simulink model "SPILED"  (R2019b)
settings: Solver=FixedStepDiscrete  StartTime=0.0  StopTime=inf  FixedStep=0.001  RelTol=1e-3  EnableMultiTasking=on
libraries: c2837xDlib x2, demo_controls x1, simulink x1, c280xlib x1

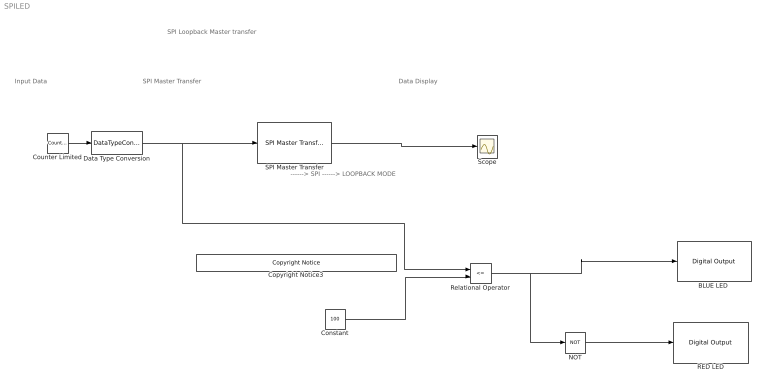
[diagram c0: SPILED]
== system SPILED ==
  note: SPI Loopback Master transfer
  note: Input Data
  note: SPI Master Transfer
  note: ------> SPI ------> LOOPBACK MODE
  note: Data Display
  "BLUE LED " : c2837xDlib/Digital Output  GPIO_Number=GPIO24~GPIO31  GPIO_Bit0=off  GPIO_BIT0_Toggle=off  GPIO_Bit1=off  GPIO_BIT1_Toggle=off  GPIO_Bit2=off  GPIO_BIT2_Toggle=off  GPIO_Bit3=off  GPIO_BIT3_Toggle=off  GPIO_Bit4=off  GPIO_BIT4_Toggle=off  GPIO_Bit5=off  GPIO_BIT5_Toggle=off  GPIO_Bit6=off  GPIO_BIT6_Toggle=off  GPIO_Bit7=on  GPIO_BIT7_Toggle=off
  Constant : Constant  Value=100
  Copyright Notice3 : demo_controls/Copyright Notice  year=2017  prod=tic2000
  Counter Limited : simulink/Sources/Counter Limited  uplimit=127  tsamp=0.1
  Data Type Conversion : DataTypeConversion  OutDataTypeStr=uint16
  NOT : Logic  Operator=NOT  IconShape=distinctive  AllPortsSameDT=off  OutDataTypeStr=boolean
  RED LED : c2837xDlib/Digital Output  GPIO_Number=GPIO32~GPIO39  GPIO_Bit0=off  GPIO_BIT0_Toggle=off  GPIO_Bit1=off  GPIO_BIT1_Toggle=off  GPIO_Bit2=on  GPIO_BIT2_Toggle=off  GPIO_Bit3=off  GPIO_BIT3_Toggle=off  GPIO_Bit4=off  GPIO_BIT4_Toggle=off  GPIO_Bit5=off  GPIO_BIT5_Toggle=off  GPIO_Bit6=off  GPIO_BIT6_Toggle=off  GPIO_Bit7=off  GPIO_BIT7_Toggle=off
  Relational Operator : RelationalOperator  Operator=<=  OutDataTypeStr=boolean  RndMeth=Simplest
  SPI Master Transfer : c280xlib/SPI Master Transfer  SPISelect=SPI_B  ClockPolarity=Falling_edge  ClockPhase=No_delay  SPIModule=uint32(0)  Mode=Master  BusSpeed=uint32(1000000)  FirstBitToTransfer=Most significant bit (MSB)  ClockMode=0  BlockFunction=Transfer  EnableRegisterAddress=off  RegisterAddress=0  OutputDataType=int8  OutputDataLength=1  DataBits=16  UseCustomSSPin=Provided by the SPI peripheral  ActiveLowSSPin=Active low  Pin=65
  Scope : Scope
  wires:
  Counter Limited/1 -> Data Type Conversion/1
  SPI Master Transfer/1 -> Scope/1
  Data Type Conversion/1 -> Relational Operator/1, SPI Master Transfer/1
  NOT/1 -> RED LED/1
  Constant/1 -> Relational Operator/2
  Relational Operator/1 -> NOT/1, "BLUE LED "/1
